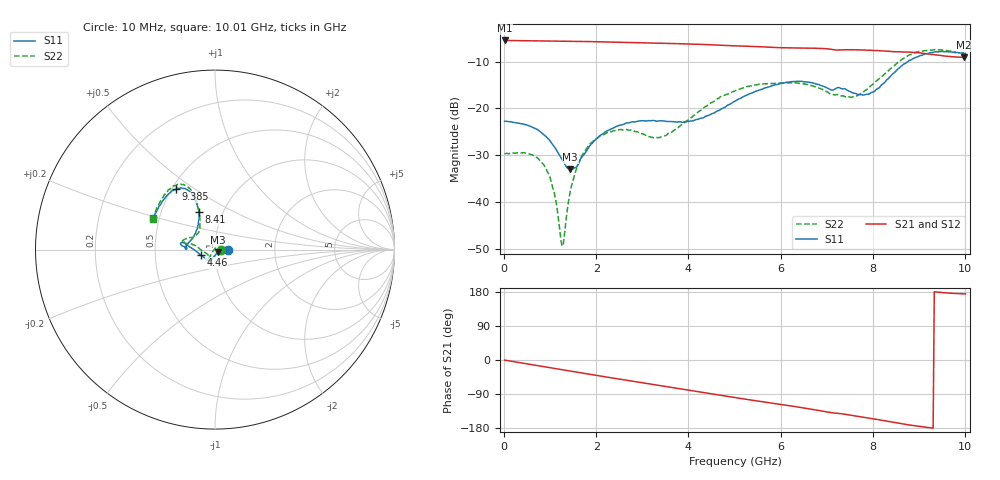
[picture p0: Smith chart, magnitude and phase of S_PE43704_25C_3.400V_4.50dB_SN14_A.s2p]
! Device ID: PE43704
! Dir: z:\PE43704\PE43704_Char_1_20130516\PE43704\AMB\3p400V\4p50dB
! Serial: 14
! Insertion: A
! Impedance: 50 ohm
! Temp: Amb
! VDD: 3.400V
! Attenuation Step: 4.50dB
! IDD: 1.140438e-01mA
#  Hz  S  RI  R  50
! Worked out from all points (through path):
!   401 points, 10 MHz to 10.01 GHz, reference 50 ohm
!   highest |S21| = -5.50 dB at 10 MHz (marker M1); lowest = -9.1 dB at 9.985 GHz (marker M2)
!   group delay of S21, straight-line fit = 53 ps
!   lowest |S11| = -32.9 dB at 1.435 GHz (marker M3), VSWR 1.05, Z = 51.7 - j1.52 ohm
!   |S11| at or under -10 dB: start of sweep to 8.763 GHz
!   |S22| runs from -49.4 to -7.5 dB; largest |S21 - S12| = 0.004
!   S11 on the Smith chart (normalised r, x): 10 MHz: 1.16, +0.00; 4.46 GHz: 0.85, -0.05; 8.41 GHz: 0.77, +0.34; 9.385 GHz: 0.52, +0.42; 10.01 GHz: 0.46, +0.19
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1e7  0.0729 9.42e-05  0.5308 -0.00221  0.5311 -0.00201  0.033 0.000389
5.6e8  0.063 0.0152  0.5161 -0.105  0.516 -0.1049  0.0262 0.0194
8.6e8  0.0509 0.0135  0.5003 -0.1581  0.5003 -0.158  0.0171 0.0183
1.06e9  0.0402 0.00651  0.4874 -0.1926  0.4874 -0.1923  0.00784 0.0116
1.26e9  0.0282 -0.0035  0.4708 -0.2262  0.4709 -0.226  -0.0022 0.00259
1.31e9  0.0249 -0.00659  0.4663 -0.234  0.4665 -0.2339  -0.00459 -0.000536
1.435e9  0.0171 -0.0147  0.4548 -0.2536  0.4546 -0.2535  -0.0104 -0.00805
1.685e9  0.00277 -0.03  0.4288 -0.2915  0.4289 -0.2913  -0.0203 -0.0235
1.935e9  -0.00863 -0.043  0.3996 -0.3259  0.3996 -0.3257  -0.0271 -0.036
2.36e9  -0.0215 -0.0575  0.3438 -0.377  0.344 -0.377  -0.0345 -0.0457
3.36e9  -0.0351 -0.0647  0.1922 -0.4575  0.1927 -0.4572  -0.0402 -0.0277
4.46e9  -0.0802 -0.0292  0.0103 -0.4785  0.0108 -0.4788  -0.1101 0.0232
5.01e9  -0.1193 0.00118  -0.0744 -0.4597  -0.0742 -0.4599  -0.1507 0.0314
5.985e9  -0.1799 0.0401  -0.2023 -0.3964  -0.2003 -0.3967  -0.1806 0.0477
6.685e9  -0.1864 0.0232  -0.2841 -0.335  -0.2842 -0.3345  -0.164 0.06
7.585e9  -0.1372 0.0488  -0.3542 -0.2303  -0.3536 -0.2301  -0.0911 0.0984
7.96e9  -0.106 0.102  -0.3753 -0.1809  -0.3756 -0.1822  -0.0843 0.1534
8.36e9  -0.0887 0.1946  -0.387 -0.123  -0.3866 -0.1249  -0.0935 0.2407
8.41e9  -0.0904 0.2087  -0.3879 -0.1155  -0.3878 -0.1169  -0.0995 0.2535
9.385e9  -0.219 0.3367  -0.3713 0.00424  -0.3719 0.00507  -0.2413 0.345
9.985e9  -0.3376 0.1841  -0.3483 0.0332  -0.3497 0.0344  -0.341 0.1769
1.001e10  -0.3429 0.1736  -0.3492 0.0337  -0.3517 0.0339  -0.3444 0.1682
